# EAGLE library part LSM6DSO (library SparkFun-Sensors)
The LSM6DSO is a system-in-package featuring a high-performance 3-axis digital accelerometer and 3-axis digital gyroscope.
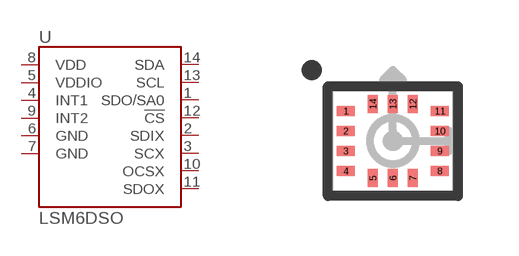
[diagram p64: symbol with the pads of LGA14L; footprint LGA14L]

Designator prefix U

## LSM6DSO (PROD_ID: IC-15837; VALUE: LSM6DS0)  [LGA14L]
1  SDO/SA0
2  SDIX
3  SCX
4  INT1
5  VDDIO
6  GND
7  GND
8  VDD
9  INT2
10  OCSX
11  SDOX
12  !CS!
13  SCL
14  SDA

## Footprint LGA14L (pad centres in mm)
Physical Chracteristics 2.5mm x 3mm Package size 14 pins 0.5mm pitch
smd 0.45 x 0.25: 1 -1.175,0.75; 2 -1.175,0.25; 3 -1.175,-0.25; 4 -1.175,-0.75; 8 1.175,-0.75; 9 1.175,-0.25; 10 1.175,0.25; 11 1.175,0.75
smd 0.25 x 0.45: 5 -0.5,-0.925; 6 0,-0.925; 7 0.5,-0.925; 12 0.5,0.925; 13 0,0.925; 14 -0.5,0.925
